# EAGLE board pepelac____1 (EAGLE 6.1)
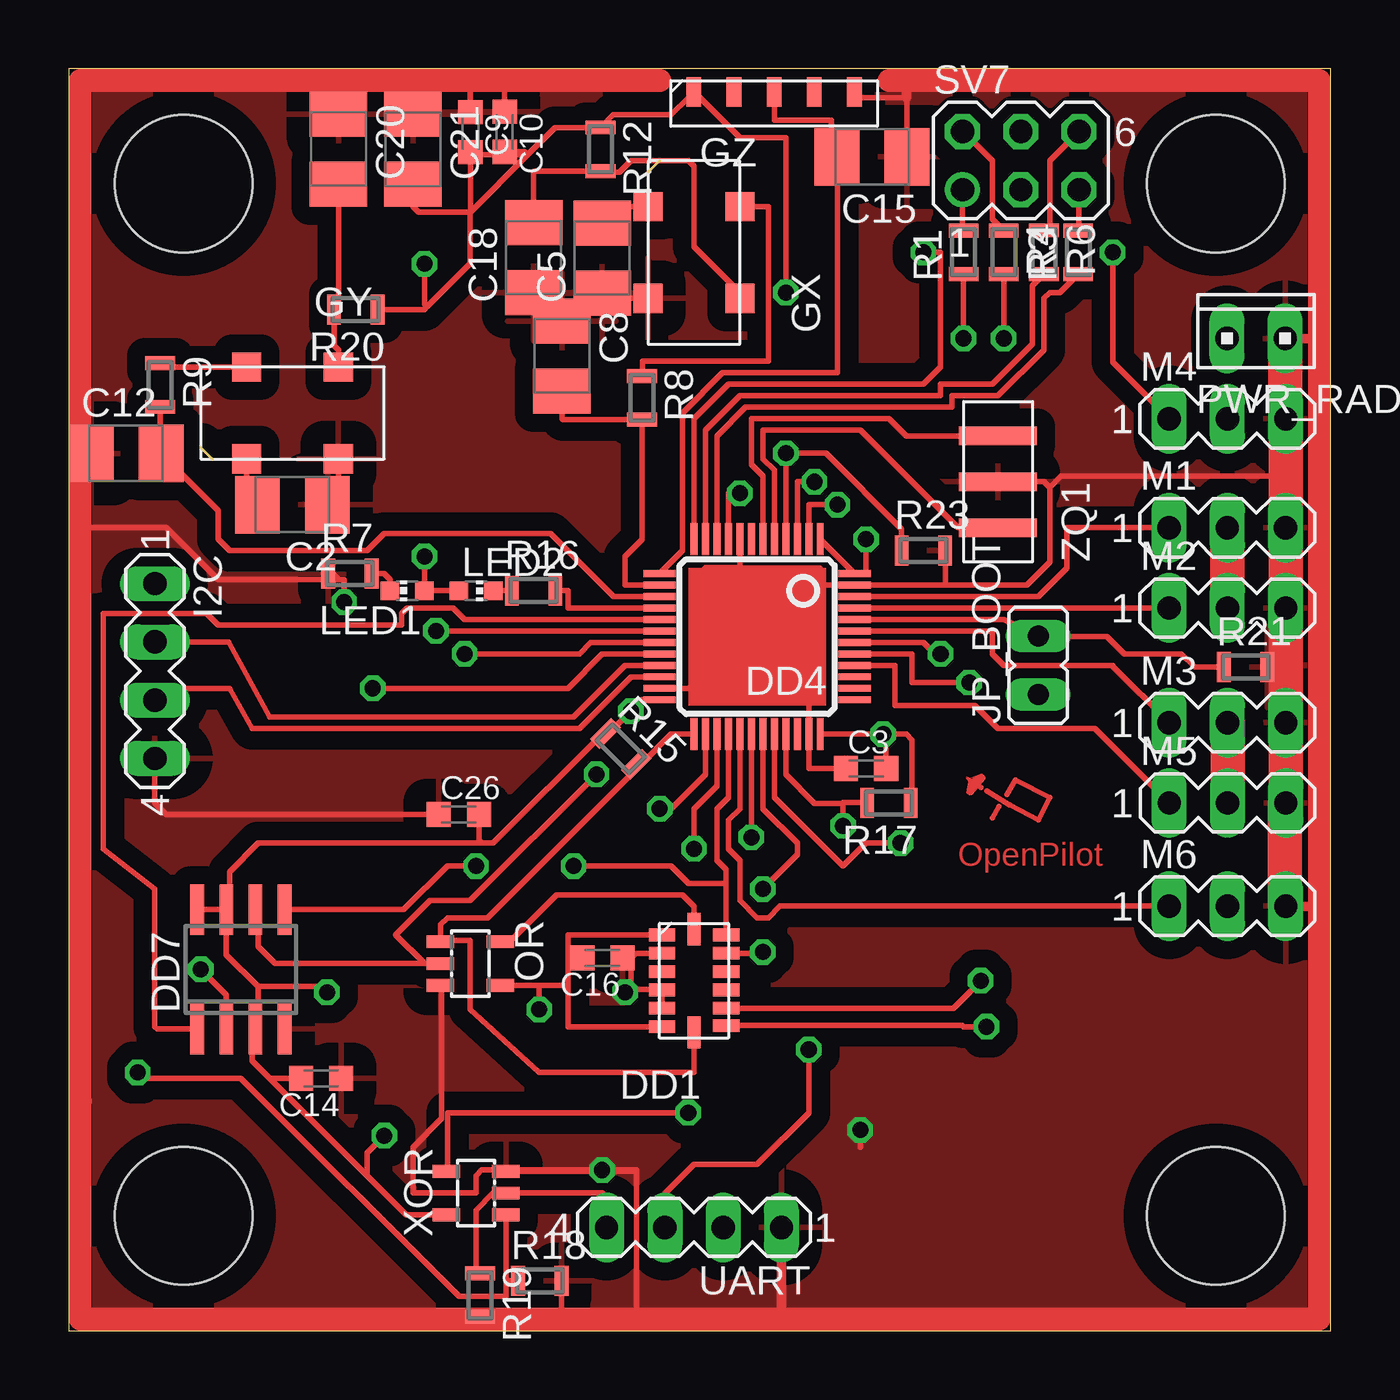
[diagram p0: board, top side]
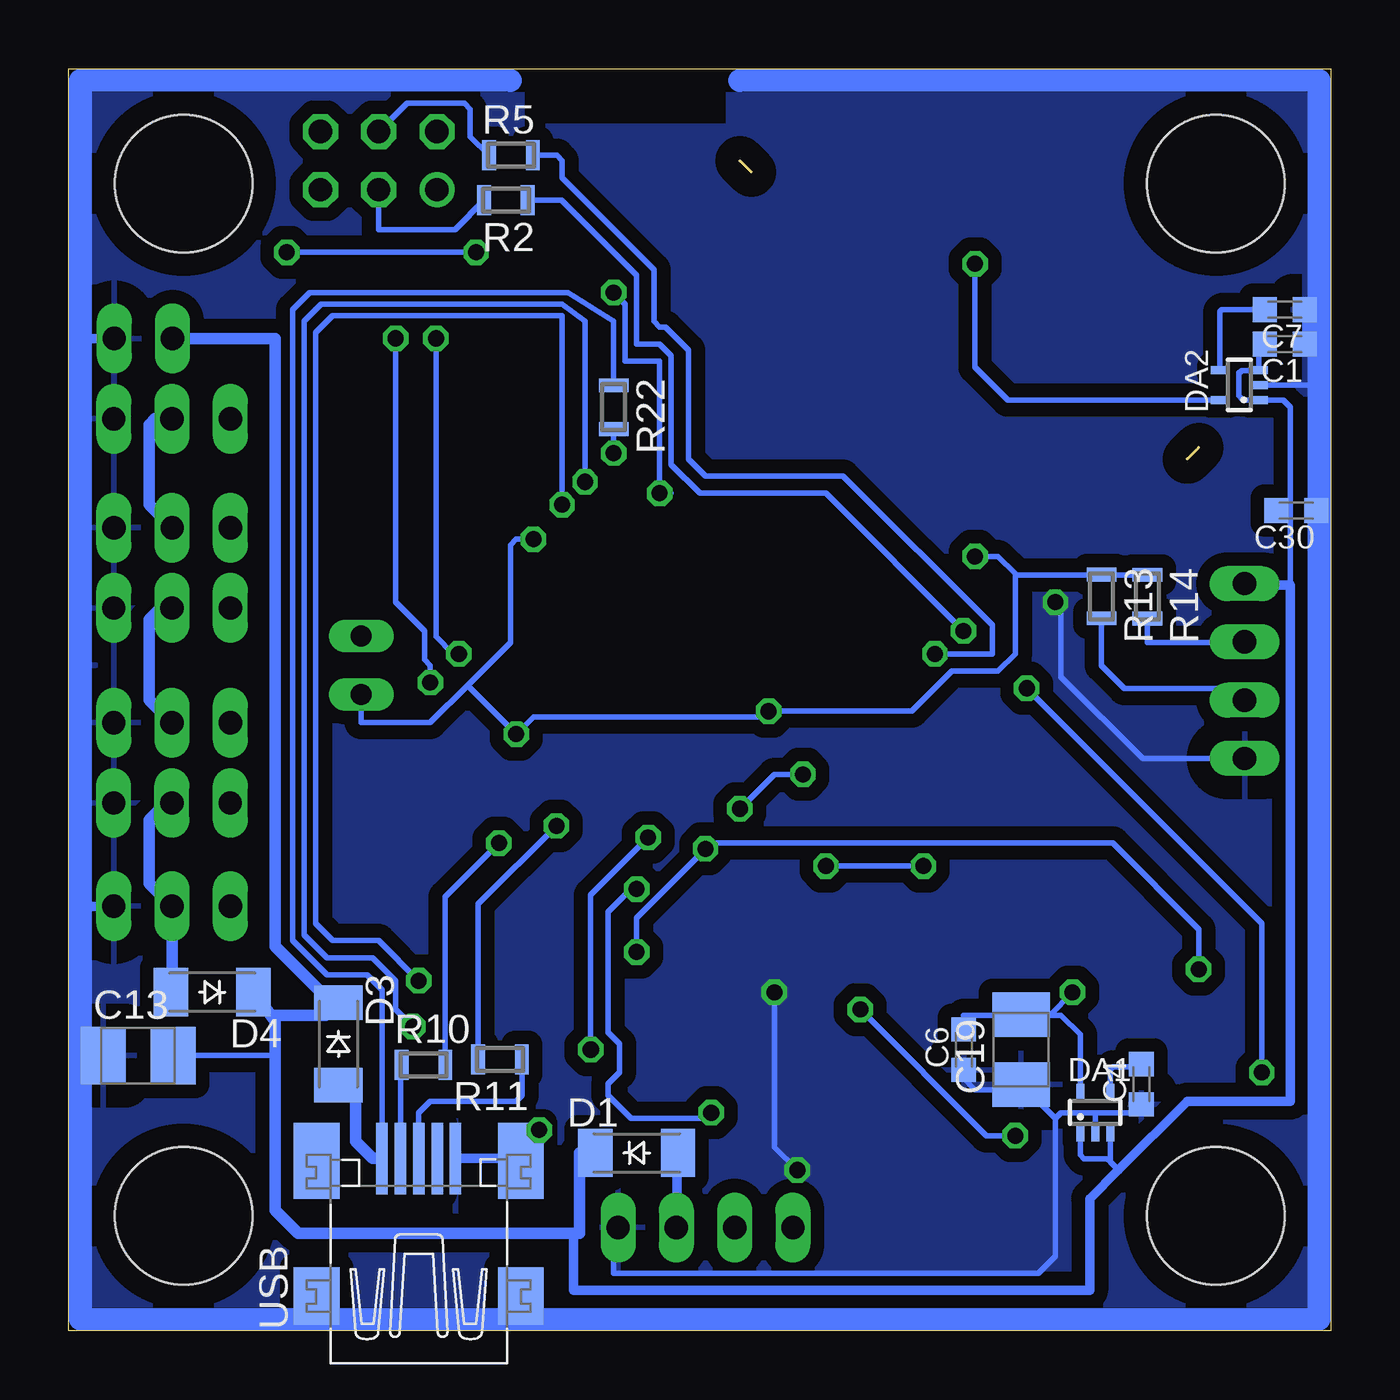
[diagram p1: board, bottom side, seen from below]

Size 55 x 55 mm. Coordinates in mm from the lower left corner, seen from the top.
Outline: 0,0 55,0 55,55 0,55 0,0
Copper layers (1*16): Top 0.035mm / dielectric 1.5mm / Bottom 0.035mm
Design rules: minimum track width 6mil, minimum drill 30mil, track to track 6mil, track to pad 6mil, pad to pad 8mil, via to via 8mil, smd to smd 8mil, copper to edge 40mil, drill to drill 8mil, minimum pad ring 10mil, minimum via ring 8mil, stop-mask expansion 4mil, vias tented up to drill 0mil, thermal gap 40mil
Holes 6 mm at 5,50 5,5 50,5 50,50

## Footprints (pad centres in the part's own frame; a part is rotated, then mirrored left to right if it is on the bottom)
C0603K = smd 1.05 x 1.08: 1 -0.875,0; 2 0.875,0
B/3528-21R = smd 1.95 x 2.5: + 1.525,0; - -1.525,0
SOD-123_MINI-SMA = smd 1.5 x 2.1: A 1.8,0; C -1.8,0
SC70-5L = smd 0.35 x 0.8: 1 -0.65,-0.85; 2 0,-0.85; 3 0.65,-0.85; 4 0.65,0.85; 5 -0.65,0.85
ACC = smd 1.145 x 0.55: 1 -1.4,2; 2 -1.4,1.2; 3 -1.4,0.4; 4 -1.4,-0.4; 5 -1.4,-1.2; 6 -1.4,-2; 8 1.4,-1.95; 9 1.4,-1.2; 10 1.4,-0.4; 11 1.4,0.4; 12 1.4,1.2; 13 1.4,2 | smd 0.55 x 1.4: 7 0,-2.25; 14 0,2.25
LQFP48 = smd 0.3 x 1.4: 1 -2.75,-4.25; 2 -2.25,-4.25; 3 -1.75,-4.25; 4 -1.25,-4.25; 5 -0.75,-4.25; 6 -0.25,-4.25; 7 0.25,-4.25; 8 0.75,-4.25; 9 1.25,-4.25; 10 1.75,-4.25; 11 2.25,-4.25; 12 2.75,-4.25; 25 2.75,4.25; 26 2.25,4.25; 27 1.75,4.25; 28 1.25,4.25; 29 0.75,4.25; 30 0.25,4.25; 31 -0.25,4.25; 32 -0.75,4.25; 33 -1.25,4.25; 34 -1.75,4.25; 35 -2.25,4.25; 36 -2.75,4.25 | smd 1.4 x 0.3: 13 4.25,-2.75; 14 4.25,-2.25; 15 4.25,-1.75; 16 4.25,-1.25; 17 4.25,-0.75; 18 4.25,-0.25; 19 4.25,0.25; 20 4.25,0.75; 21 4.25,1.25; 22 4.25,1.75; 23 4.25,2.25; 24 4.25,2.75; 37 -4.25,2.75; 38 -4.25,2.25; 39 -4.25,1.75; 40 -4.25,1.25; 41 -4.25,0.75; 42 -4.25,0.25; 43 -4.25,-0.25; 44 -4.25,-0.75; 45 -4.25,-1.25; 46 -4.25,-1.75; 47 -4.25,-2.25; 48 -4.25,-2.75
SOIC8 = smd 0.6 x 2.2: 1 -1.905,-2.6; 2 -0.635,-2.6; 3 0.635,-2.6; 4 1.905,-2.6; 5 1.905,2.6; 6 0.635,2.6; 7 -0.635,2.6; 8 -1.905,2.6
GIRO = smd 1.27 x 1.27: 1 1,2; 2 -3,2; 3 -3,-2; 4 1,-2
GZ = smd 0.635 x 1.27: 1 -3.5,0.5; 2 -1.75,0.5; 3 0,0.5; 4 1.75,0.5; 5 3.5,0.5
MA04-1 = drill 1.016 long: 1 -3.81,0; 2 -1.27,0; 3 1.27,0; 4 3.81,0
JP1 = drill 0.914 long: 1 0,-1.27; 2 0,1.27
CHIP-LED0603 = smd 0.8 x 0.8: A 0,-0.75; C 0,0.75
MA03-1 = drill 1.016 long: 1 -2.54,0; 2 0,0; 3 2.54,0
SOT23-5L = smd 0.55 x 1.2: 1 -0.95,-1.3; 2 0,-1.3; 3 0.95,-1.3; 4 0.95,1.3; 5 -0.95,1.3
10X02MTA = drill 1.016 long: 1 1.27,0; 2 -1.27,0
MINI_MELF-0102W = smd 0.6 x 1.3: 1 -0.95,0; 2 0.95,0
MA03-2 = drill 1.016: 1 -2.54,-1.27 | drill 1.016 octagon: 2 -2.54,1.27; 3 0,-1.27; 4 0,1.27; 5 2.54,-1.27; 6 2.54,1.27
32005-400 = smd 3.1 x 0.5: 1 3,1.6; 2 3,0.8; 3 3,0; 4 3,-0.8; 5 3,-1.6 | smd 2.5 x 2: M1 -3,-4.45; M2 -3,4.45 | smd 3.3 x 2: M3 2.9,4.45; M4 2.9,-4.45
QARZ = smd 0.8 x 3.4: 1 -2,0; 2 0,0; 3 2,0

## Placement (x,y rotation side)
C1  [C0603K]  2,43 180 bottom
C2  [B/3528-21R]  9.75,36 180 top
C3  [C0603K]  34.75,24.5 0 top
C4  [C0603K]  8.26,10.74 90 bottom
C5  [B/3528-21R]  23.25,46.75 90 top
C6  [C0603K]  15.99,12.25 90 bottom
C7  [C0603K]  2,44.5 180 bottom
C8  [B/3528-21R]  21.49,42.48 270 top
C9  [C0603K]  17.5,52.24 270 top
C10  [C0603K]  19,52.25 270 top
C12  [B/3528-21R]  2.5,38.24 0 top
C13  [B/3528-21R]  51.98,11.99 0 bottom
C14  [C0603K]  11,11 180 top
C15  [B/3528-21R]  35.01,51.16 180 top
C16  [C0603K]  23.25,16.25 180 top
C18  [B/3528-21R]  20.26,46.77 90 top
C19  [B/3528-21R]  13.5,12.25 90 bottom
C20  [B/3528-21R]  11.75,51.5 270 top
C21  [B/3528-21R]  15,51.49 270 top
C26  [C0603K]  17,22.5 0 top
C30  [C0603K]  1.5,35.75 180 bottom
D1  CGRM4001-G  [SOD-123_MINI-SMA]  30.25,7.75 0 bottom
D3  CGRM4001-G  [SOD-123_MINI-SMA]  43.25,12.5 270 bottom
D4  CGRM4001-G  [SOD-123_MINI-SMA]  48.75,14.75 180 bottom
DA1  [SC70-5L]  10.26,9.51 0 bottom
DA2  [SC70-5L]  3.98,41.22 90 bottom
DD1  [ACC]  27.25,15.25 0 top
DD4  [LQFP48]  30,30.25 180 top
DD7  [SOIC8]  7.5,15.75 0 top
GX  [GIRO]  27.25,47.99 90 top
GY  [GIRO]  8.75,40 180 top
GZ  [GZ]  30.74,53.49 0 top
I2C  [MA04-1]  3.75,28.75 270 top
JP_BOOT  [JP1]  42.25,29 0 top
LED1  [CHIP-LED0603]  14.75,32.25 90 top
LED2  [CHIP-LED0603]  17.75,32.25 270 top
M1  [MA03-1]  50.5,35 0 top
M2  [MA03-1]  50.5,31.5 0 top
M3  [MA03-1]  50.5,26.5 0 top
M4  [MA03-1]  50.5,39.75 0 top
M5  [MA03-1]  50.51,23 0 top
M6  [MA03-1]  50.5,18.5 0 top
OR  [SOT23-5L]  17.5,16 270 top
PWR_RADIO  [10X02MTA]  51.75,43.25 0 top
R1  [MINI_MELF-0102W]  39,47 90 top
R2  [MINI_MELF-0102W]  35.95,49.27 180 bottom
R3  [MINI_MELF-0102W]  44,47 90 top
R4  [MINI_MELF-0102W]  40.75,47 270 top
R5  [MINI_MELF-0102W]  35.73,51.23 0 bottom
R6  [MINI_MELF-0102W]  42.5,47.01 270 top
R7  [MINI_MELF-0102W]  12.25,33 0 top
R8  [MINI_MELF-0102W]  24.98,40.66 270 top
R9  [MINI_MELF-0102W]  3.98,41.22 270 top
R10  [MINI_MELF-0102W]  39.54,11.59 0 bottom
R11  [MINI_MELF-0102W]  36.21,11.83 180 bottom
R12  [MINI_MELF-0102W]  23.17,51.49 270 top
R13  [MINI_MELF-0102W]  9.99,32 270 bottom
R14  [MINI_MELF-0102W]  8,31.99 270 bottom
R15  [MINI_MELF-0102W]  24.06,25.36 315 top
R16  [MINI_MELF-0102W]  20.26,32.25 0 top
R17  [MINI_MELF-0102W]  35.75,23 180 top
R18  [MINI_MELF-0102W]  20.53,2.17 0 top
R19  [MINI_MELF-0102W]  17.92,1.55 270 top
R20  [MINI_MELF-0102W]  12.51,44.5 180 top
R21  [MINI_MELF-0102W]  51.29,28.92 0 top
R22  [MINI_MELF-0102W]  31.25,40.25 270 bottom
R23  [MINI_MELF-0102W]  37.25,34 0 top
SV7  [MA03-2]  41.49,51 0 top
UART  [MA04-1]  27.25,4.5 180 top
USB  MINI-USB_SHIELD5P4-32005-400  [32005-400]  39.75,4.5 90 bottom
XOR  SN74LVC1G86DBVR  [SOT23-5L]  17.75,6 90 top
ZQ1  QARZ  [QARZ]  40.5,37 90 top

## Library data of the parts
C1 C3 C4 C6 C7 C9 C10 C14 C16 C26 C30 R1-R23 = resistor
C2 C5 C8 C12 C13 C15 C18-C21 = rcl
D1 D3 D4 = diode
DA1 DA2 DD1 DD4 DD7 GX GY GZ OR XOR ZQ1 = pepelac
I2C M1-M6 SV7 UART = con-lstb; OC_FARNELL: unknown; OC_NEWARK: unknown
JP_BOOT = jumper
LED1 LED2 = led
PWR_RADIO = con-amp
USB = con-cypressindustries; OC_FARNELL: unknown; OC_NEWARK: unknown

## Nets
+5V: D4.A M1.2 M2.2 M3.2 M4.2 M5.2 M6.2
GND: C1.1 C2.- C3.1 C4.1 C5.- C6.1 C7.1 C8.- C9.1 C10.1 C12.- C13.- C14.1 C15.- C16.1 C18.- C19.- C20.- C21.- C26.1 C30.1 DA1.2 DA2.2 DD1.2 DD1.4 DD1.5 DD4.8 DD4.23 DD4.35 DD4.47 DD7.4 GX.2 GY.2 GZ.5 I2C.4 M1.3 M2.3 M3.3 M4.3 M5.3 M6.3 OR.3 PWR_RADIO.1 R7.1 R18.2 R19.2 R21.2 R23.2 UART.1 USB.5 XOR.3 ZQ1.2
N$1: DD4.6 ZQ1.3
N$2: GX.4 R8.1
N$3: GY.4 R9.1
N$4: DD1.7 DD4.25 OR.1 R15.2
N$5: DD4.16 R16.2
N$6: DD4.33 R11.2 R17.2
N$7: DD4.29 M6.1
N$8: D1.A UART.2
N$9: C18.+ GX.3 R12.2
N$10: C20.+ GY.3 R20.2
N$11: DD1.9 DD4.2
N$12: LED2.C R16.1
N$13: C7.2 DA2.4
N$14: C12.+ DD4.15 R9.2
N$15: C8.+ DD4.14 R8.2
N$16: LED1.C R7.2
N$17: DD1.8 DD4.3
N$18: C2.+ GY.1
N$19: R1.2 SV7.1
N$20: R2.2 SV7.3
N$21: R3.2 SV7.5
N$22: R4.1 SV7.2
N$23: R5.1 SV7.4
N$24: R6.1 SV7.6
N$25: DD4.42 R1.1
N$26: DD4.41 R4.2
N$27: DD4.18 R2.1
N$28: DD4.19 R5.2
N$29: DD4.10 R3.1
N$30: DD4.11 R6.2
N$31: C15.+ DD4.13 GZ.3
N$32: DD4.5 ZQ1.1
N$34: DD4.46 M1.1
N$35: DD4.45 M2.1
N$36: DD4.43 M3.1
N$37: DD4.40 M5.1
N$38: DD4.12 M4.1
N$39: C5.+ GX.1
N$40: R19.1 UART.4 XOR.2
N$41: C4.2 DA1.4
N$43: DD4.30 UART.3
N$44: DD4.4 R22.2 R23.1
N$45: D3.A R22.1 USB.1
N$46: R10.1 USB.2
N$47: R11.1 USB.3
N$48: DD4.20 R18.1 XOR.1
N$49: DD4.31 XOR.4
N$50: DD4.22 I2C.3 R13.2
N$51: DD4.21 I2C.2 R14.2
N$53: DD4.32 R10.2
N$54: DD4.44 JP_BOOT.2 R21.1
N$58: DD4.17 DD7.1
N$60: DD4.26 DD7.6 OR.2
N$61: DD1.12 DD4.27 DD7.2
N$62: DD1.14 OR.5
N$63: DD1.13 DD4.28 DD7.5
V+: C1.2 C13.+ C30.2 D1.C D3.C D4.C DA1.1 DA1.3 DA2.1 DA2.3 PWR_RADIO.2
VCC: C9.2 C10.2 C21.+ DA2.5 DD4.9 GZ.1 R12.1 R20.1
VDD: C3.2 C6.2 C14.2 C16.2 C19.+ C26.2 DA1.5 DD1.1 DD1.6 DD4.1 DD4.24 DD4.36 DD4.48 DD7.3 DD7.7 DD7.8 JP_BOOT.1 LED1.A LED2.A OR.4 R13.1 R14.1 R15.1 R17.1 XOR.5

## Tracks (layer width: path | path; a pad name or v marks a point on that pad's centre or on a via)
+5V  (via drill 0.7)
  Top 0.5: M3.2
  Top 1.5: M4.2 | M1.2 M2.2 M1.2 | M3.2 M5.2
  Bottom 0.5: M4.2 51.25,39.75 51.5,39.5 51.5,36 M1.2 | M2.2 51,31.5 51.5,31 51.5,27.5 M3.2 | M5.2 50.75,23 51.5,22.25 51.5,19.5 M6.2 50.5,14.8 D4.A
  other vias: 50.5,31.5
GND  (via drill 0.7)
  Top 0.25: ZQ1.2 42.5,37 42.75,36.75 | 42.75,36.75 42.75,33.5 41.75,32.5 39.75,32.5 | 39.75,32.5 DD4.47 32.75,32.5 | 42.75,36.75 43.25,37.25 53,37.25 53,35 | 32.75,32.5 32.75,33.25 29.25,33.25 | 29.25,33.25 DD4.8 | DD4.23 27,28 27.25,28.25 27.25,32.75 27.75,33.25 29.25,33.25 | 32.75,32.5 32.25,32.5 DD4.35 32.25,24.5 | GZ.5 34.48,53.75 36.5,53.75 36.53,53.72 C15.- | DD1.2 24.7,16.45 24.5,16.25 | 24.5,16.25 24.5,15 | 24.5,15 24.5,14.99 24.61,14.88 25.82,14.88 DD1.4 | DD1.4 DD1.5 DD1.4 | 0.75,10.25 0.5,10 | R23.2 38.2,32.55 38.25,32.5 39.75,32.5 | 39.75,32.5 | 24.5,15 v24.25,14.75 24.38,14.88 26.05,14.88 26,14.93 26,15 DD1.4 | XOR.3 24.7,6.95 24.75,7 | 24.75,7 24.75,0.5 | 24.75,7 v23.25,7 18,7 17.75,6.75 17.75,6 15,6 15,8 16.25,9.25 16.25,15 OR.3 | 12,37.75 GY.2 | v34.5,8.75 34.5,8 | R19.2 18.9,0.6 19,0.5 | R21.2 52.96,28.92 53.04,29 | GX.2 23.47,44.99 C5.- 22.71,45.22 C8.- C18.- | v12,31.75 12,32.75 11.75,32.75 | 11.75,32.75 6.5,32.75 4.25,35 0.5,35 | C12.- 0.51,38.24 0.5,38.25 | C2.- 11.5,36 11.75,36.25 GY.2 | C21.- 15,54.25 17.5,54.25 C9.1 | 17.5,53 C9.1 | C9.1 | R7.1 11.5,33 11.75,32.75 | R18.2 21.48,0.77 21.75,0.5 | C3.1 32.25,24.5 | 32.25,24.5 | C10.1 19,54.25 19.25,54.5 | C16.1 24.5,16.25 | C26.1 4.25,22.5 3.75,23 3.75,25
  Top 0.406: 36.5,53.75 36.5,54.5 | 35.75,54.5 54.5,54.5 54.5,43.5 54.25,43.25 v53,43.25 | UART.1 31.06,0.69 31.25,0.5 | 53.25,18.5 54.5,18.5
  Top 1: 35.75,54.5 36.5,54.5 54.5,54.5 54.5,18.5 54.5,0.5 31.25,0.5 24.75,0.5 21.75,0.5 19,0.5 0.5,0.5 0.5,10 0.5,35 0.5,38.25 0.5,54.5 19.25,54.5 25.75,54.5
  Top 1.5: M6.3 53,18.5 53,23 | M5.3 M3.3 53.04,29 M2.3 M1.3 | 53,35 M1.3 M4.3 53.02,39.75 PWR_RADIO.1
  Bottom 0.25: v24.25,14.75 24.25,8 v23.25,7 | I2C.4 8.19,24.94 11.75,28.5 11.75,31.25 v12,31.75 | 35.5,7.5 34.5,7.5 v34.5,8.75 | DA2.2 0.53,41.22 0.5,41.25 | DA1.2 10.26,9.49 10.25,9.5 | 10.25,9.5 11.75,9.5 12,9.25 | 12,9.25 12,3.25 12.75,2.5 31.25,2.5 31.25,4.25 31,4.5 | C4.1 8.38,9.87 8.75,9.5 10.25,9.5 | C30.1 0.5,35.75 | 12,9.25 13.48,10.73 C19.- 13.73,10.5 15.5,10.5 15.99,10.99 C6.1 | C13.- 54.49,11.99 54.5,12 | C7.1 C1.1 1,43 0.5,42.5
  Bottom 0.406: USB.5 35.5,7.5 | v53,43.25 54.5,43.25 | 53,18.5 54.5,18.5
  Bottom 1: 35.75,54.5 54.5,54.5 54.5,43.25 54.5,18.5 54.5,12 54.5,0.5 0.5,0.5 0.5,35.75 0.5,41.25 0.5,42.5 0.5,54.5 25.75,54.5
  pour Top (isolate 0.8): 0,55 26.25,55 26.25,54.75 26.25,52.5 35.25,52.5 35.25,55 55,55 55,0 0,0
  pour Bottom (isolate 0.6): 26.25,55 26.25,52.5 35.25,52.5 35.25,55 55,55 55,0 0,0 0,55
N$1
  Top 0.25: DD4.6 30.25,36 30.25,37.25 29.75,37.75 29.75,39.75 35.75,39.75 36.5,39 ZQ1.3 | 40.75,39 ZQ1.3 | ZQ1.3
N$2
  Top 0.152: 25,41.75 R8.1
  Top 0.25: GX.4 30.5,48.99 30.5,49 30.5,42.25 25,42.25 25,41.75 25,41.5
N$3
  Top 0.25: GY.4 4.15,42 R9.1
N$4
  Top 0.25: DD1.7 27.25,11.25 20.5,11.25 17.5,14 17.5,17 16.25,17 OR.1 16.2,17.7 16.5,18 18.25,18 24.94,24.69 | DD4.25 26.25,26 24.94,24.69 | R15.2 24.94,24.69
N$5
  Top 0.152: 21.25,32.25 R16.2
  Top 0.25: DD4.16 21.75,31.5 21.75,32.25 21.25,32.25
N$6  (via drill 0.7)
  Top 0.25: v33.75,22 33.75,23.02 | DD4.33 31.25,24.25 32.49,22.99 33.72,22.99 33.75,23.02 | 33.75,23.02 34.78,23.02 R17.2
  Bottom 0.25: R11.2 37.16,18.59 v33.75,22
N$7
  Top 0.25: M6.1 31,18.5 30.5,18 30,18 29.25,18.75 29.25,20.5 28.75,21 28.75,22.25 29.25,22.75 DD4.29
N$8
  Bottom 0.152: 28.5,7.75 D1.A
  Bottom 0.406: UART.2 28.5,4.5 28.5,7.75
N$9
  Top 0.25: GX.3 29.25,45.25 27.25,47.25 27.25,50.75 27,51 24.5,51 24,50.5 23.21,50.5 R12.2 20.29,50.54 20.25,50.5 20.25,48.3 C18.+
N$10
  Top 0.152: 11.5,44.5 R20.2
  Top 0.25: R20.2 11.56,42.94 11.75,42.75 GY.3 | C20.+ 11.75,44.75 11.5,44.5
N$11  (via drill 0.7)
  Top 0.25: DD4.2 32.25,36 v33.5,36 | v39.75,15.25 38.55,14.05 DD1.9
  Bottom 0.25: v33.5,36 33.5,44.25 43.5,44.25 44.25,43.5 44.25,17.75 43.5,17 41.5,17 v39.75,15.25
N$12
  Top 0.25: LED2.C R16.1
N$13
  Bottom 0.152: 3,44.5 C7.2
  Bottom 0.25: DA2.4 4.83,44.42 4.75,44.5 3,44.5
N$14
  Top 0.25: R9.2 3.98,38.28 C12.+ 4.02,38.23 6.5,35.75 6.5,34.5 7,34 13,34 13.75,34.75 21,34.75 23.75,32 DD4.15
N$15
  Top 0.25: C8.+ 21.5,39.75 21.54,39.71 R8.2 24.98,34.48 24.25,33.75 24.25,32.5 DD4.14
N$16
  Top 0.152: LED1.C
  Top 0.25: R7.2 13.75,33 14,32.75 LED1.C
N$17  (via drill 0.7)
  Top 0.25: DD4.3 31.75,36 31.75,37 v32.5,37 | v40,13.25 39,13.25 38.95,13.3 DD1.8
  Bottom 0.25: v32.5,37 32.5,44 33.5,44.75 44,44.75 44.75,44 44.75,17.25 43.75,16.25 41.75,16.25 40.75,15.25 40.75,14 v40,13.25
N$18
  Top 0.25: C2.+ 7.75,36 GY.1
N$19
  Top 0.25: R1.2 38.95,48 SV7.1
N$20
  Bottom 0.25: R2.2 38.17,48 41.5,48 41.49,48.01 SV7.3
N$21
  Top 0.25: R3.2 44.03,47.99 SV7.5
N$22
  Top 0.25: R4.1 40.25,48.45 40.25,51 38.98,52.27 SV7.2
N$23
  Bottom 0.152: 41.5,52.25 SV7.4
  Bottom 0.25: R5.1 37.5,52.05 37.5,53.25 37.75,53.5 40.25,53.5 41.5,52.25
N$24
  Top 0.25: R6.1 42.75,48.2 42.75,51 44.02,52.27 SV7.6
N$25  (via drill 0.7)
  Top 0.25: v39,43.25 R1.1 | DD4.42 37.25,30 37.75,29.5 v38,29.5
  Bottom 0.25: v39,43.25 39,30.25 38.25,29.5 v38,29.5
N$26  (via drill 0.7)
  Top 0.152: 40.75,46 R4.2
  Top 0.25: v40.75,43.25 40.75,46 | DD4.41 36.75,29.5 36.75,28.25 v39.25,28.25
  Bottom 0.25: v40.75,43.25 40.75,31.75 39.5,30.5 39.5,29.25 39.25,29 v39.25,28.25
N$27  (via drill 0.7)
  Top 0.25: DD4.18 v16,30.5
  Bottom 0.25: R2.1 33.52,49.27 30.25,46 30.25,43 29.25,43 28.75,42.5 28.75,37.75 27.5,36.5 22,36.5 v16,30.5
N$28  (via drill 0.7)
  Top 0.25: DD4.19 22.75,30 22.25,29.5 v17.25,29.5
  Bottom 0.25: R5.2 33.73,51.23 33.5,51 33.5,50.25 29.5,46.25 29.5,44 29.25,43.75 29,43.75 28,42.75 28,38 27.25,37.25 21.25,37.25 14.75,30.75 14.75,29.5 v17.25,29.5
N$29
  Top 0.152: DD4.10
  Top 0.25: R3.1 43.2,45.25 42.75,45.25 42.5,45 42.5,42.75 40.5,40.75 38.5,40.75 38.5,40.25 29.5,40.25 28.25,39 DD4.10
N$30
  Top 0.25: R6.2 42,45.55 42,43 40.25,41.25 38,41.25 38,40.75 29.25,40.75 27.75,39.25 DD4.11 | DD4.11 27.75,34.25 | DD4.11
N$31
  Top 0.152: 30.75,53.75 GZ.3
  Top 0.25: DD4.13 26.75,34 26.75,40 28.5,41.75 33.5,41.75 33.5,51.15 | GZ.3 30.75,53.75 30.75,52.75 33.25,52.75 33.25,51.5 33.5,51.25 33.5,51.15 | C15.+ 33.5,51.15
N$32
  Top 0.25: DD4.5 30.75,36.25 30.75,37.5 30.25,38 30.25,39.25 34.5,39.25 38.75,35 ZQ1.1
N$34
  Top 0.25: M1.1 43.5,35 43.5,33.25 42.25,32 DD4.46
N$35
  Top 0.25: M2.1 48,31.5 42.75,31.5 DD4.45
N$36
  Top 0.152: DD4.43
  Top 0.25: DD4.43 40.25,30.5 40.25,29.5 40.75,29 45.5,29 45.5,28.96 M3.1
N$37
  Top 0.152: DD4.40
  Top 0.25: M5.1 44.72,26.25 40.5,26.25 39.5,27.25 36,27.25 36,29 DD4.40
N$38  (via drill 0.7)
  Top 0.152: 27.25,34.75 DD4.12
  Top 0.25: M4.1 45.5,42.21 v45.5,47 | 27.25,34.75 27.25,39.75 28.75,41.25 37.25,41.25 38,42 38,47 v37.25,47
  Bottom 0.25: v45.5,47 v37.25,47
N$39
  Top 0.25: C5.+ 23.25,48.99 23.25,49 GX.1
N$40
  Top 0.152: 18,2.5 R19.1
  Top 0.25: UART.4 23.44,5.81 23.25,6 XOR.2 | XOR.2 | XOR.2 18.5,6 17.75,5.25 17.75,2.75 18,2.5
N$41
  Bottom 0.25: DA1.4 9.61,11.39 9.5,11.5 8.25,11.5 C4.2
N$43  (via drill 0.7)
  Top 0.25: UART.3 25.98,5.98 27.25,7.25 30,7.25 32.25,9.5 v32.25,12.25 | v29.75,21.5 DD4.30
  Bottom 0.25: v32.25,12.25 32.25,19 v29.75,21.5
N$44  (via drill 0.7)
  Top 0.152: DD4.4
  Top 0.25: DD4.4 v31.25,38.25 33,38.25 36.3,34.95 R23.1
  Bottom 0.25: R22.2 v31.25,38.25
N$45
  Bottom 0.25: USB.1 41.35,14.85 42,15.5 43.75,15.5 45.25,17 45.25,44.5 44.5,45.25 33.25,45.25 31.25,44 R22.1
  Bottom 0.5: USB.1 41.75,7.5 42.5,8.25 42.5,10.75 43.2,10.75 D3.A
N$46
  Bottom 0.25: USB.2 40.55,11.53 R10.1
N$47
  Bottom 0.152: 35.25,11.75 R11.1
  Bottom 0.25: USB.3 39.75,9.5 39.25,10 35.5,10 35.25,10.25 35.25,11.75
N$48  (via drill 0.7)
  Top 0.25: DD4.20 23.5,29.5 23.25,29.5 21.75,28 v13.25,28 | XOR.1 19.05,3.8 19.06,2.23 | 19.06,2.23 19.06,1.49 17,1.5 7.5,11 3.25,11 v3,11.25 | R18.1 19.16,2.17 19.09,2.23 19.06,2.23 | 19.06,2.23
  Bottom 0.25: v3,11.25 3,17.75 v13.25,28
N$49  (via drill 0.7)
  Top 0.152: 16.5,7 XOR.4
  Top 0.25: DD4.31 30.25,22.75 31.75,21.25 31.75,20.75 v30.25,19.25 | v27,9.5 16.5,9.5 16.5,7
  Bottom 0.25: v30.25,19.25 30.5,19.25 31.5,18.25 31.5,13 31,12.5 31,11.25 31.5,10.75 31.5,10.25 30.5,9.25 27,9.25 v27,9.5
N$50
  Top 0.25: DD4.22 24.5,28.5 22.25,26.25 8,26.25 7,28 4.25,28 3.75,27.5 I2C.3
  Bottom 0.25: R13.2 9.99,28.99 9,28 3.75,28 I2C.3
N$51
  Top 0.25: DD4.21 24.25,29 22,26.75 8.75,26.75 6.98,30.02 I2C.2
  Bottom 0.152: 3.75,30 I2C.2
  Bottom 0.25: 3.79,30.04 3.75,30 8,30 R14.2
N$53  (via drill 0.7)
  Top 0.25: v36.25,21.25 34.75,21.25 33.75,20.25 30.75,23.25 DD4.32
  Bottom 0.25: R10.2 38.59,18.91 v36.25,21.25
N$54
  Top 0.152: 42.5,30.25 JP_BOOT.2
  Top 0.25: JP_BOOT.2 40.75,31 DD4.44 | R21.1 49.08,28.92 48.5,29.5 46,29.5 45.25,30.25 42.5,30.25 42.25,30.25
N$58
  Top 0.25: DD4.17 17.25,31 16.75,31.5 14.75,31.5 14.5,31.25 14.5,30.75 6.5,30.75 6,31.25 1.5,31.25 1.5,21 3.75,19.25 3.75,13.25 3.85,13.15 DD7.1
N$60  (via drill 0.7)
  Top 0.25: v23,24.25 17.5,18.75 15.75,18.75 14.25,17.25 15.5,16 OR.2 9,16 8.25,16.75 8.25,18.23 DD7.6 | v25.75,22.75 26.25,22.75 27.75,24.25 DD4.26
  Bottom 0.25: v23,24.25 24.25,24.25 v25.75,22.75
N$61  (via drill 0.7)
  Top 0.25: DD1.12 30.2,16.45 v30.25,16.5 | v27.25,21 27.25,22.75 28.25,23.75 DD4.27 | DD7.2 6.86,14.64 v5.75,15.75
  Bottom 0.25: v30.25,16.5 30.25,18 v27.25,21 27,21.25 9.5,21.25 5.75,17.5 v5.75,15.75
N$62
  Top 0.25: OR.5 19.2,16.95 21.25,19 26.75,19 27.25,18.5 DD1.14
N$63  (via drill 0.7)
  Top 0.25: DD1.13 28.65,19.5 | 28.65,19.5 28.65,20.1 28.25,20.5 28.25,22.75 28.75,23.25 DD4.28 | DD7.5 14.6,18.35 16.5,20.25 v17.75,20.25 | v22,20.25 26.25,20.25 27,19.5 28.65,19.5
  Bottom 0.25: v17.75,20.25 v22,20.25
S$1
  Top 0.25: 40.88,23.38 41.25,24 42.75,23.25 42.25,22.25 41.01,22.91
S$2
  Top 0.25: 39.75,23.68 39.36,23.95 39.55,23.83 39.78,24.13 39.44,23.99 39.35,23.89 39.26,23.51 39.26,23.5 39.62,23.92 39.84,24.09 39.32,23.45 39.5,24 39.5,23.75
S$3
  Top 0.09: 39.25,24 39.18,24.08 39.24,24.05 39.25,24
S$4
  Top 0.03: 39.91,24.17 39.79,24.26 39.24,24.04 39.13,23.45 39.26,23.36
S$5
  Top 0.03: 39.11,24.12 39.22,23.96 39.3,24.07 39.12,24.13
S$6
  Top 0.03: 39.72,23.61 39.81,23.72
S$7
  Top 0.25: 41,22.92 40.02,23.52
S$8
  Top 0.25: 40.53,22.84 40.25,22.34
V+
  Bottom 0.25: 1.75,35.75 1.75,40.25 2.07,40.57 DA2.1 3.82,40.57 4,40.75 4,41.75 3.97,41.75 3.87,41.85 3.15,41.85 DA2.3 3.13,42.75 C1.2 3,43 | 1.75,35.75 1.75,32.5 | DA1.3 9.61,7.36 | 9.61,7.36 9.25,7 | DA1.1 10.91,7.66 10.75,7.5 9.75,7.5 9.61,7.36 | C13.+ 46.01,11.99 46,12 | C30.2 1.75,35.75
  Bottom 0.406: 3.75,32.5 1.75,32.5 1.75,10 6.25,10 9.25,7 10.5,5.75 10.5,1.75 33,1.75 33,4.25
  Bottom 0.5: D1.C 32.75,7.75 32.75,4.25 33,4.25 45,4.25 46,5.25 46,12 46,13.5 | 46,13.5 46,13.75 43.8,13.75 D3.C 43.25,14.25 43.5,14.25 46,16.75 46,43.25 PWR_RADIO.2 | D4.C 46,13.5
VCC  (via drill 0.7)
  Top 0.152: 27,53.75 GZ.1
  Top 0.25: DD4.9 28.75,36.5 v29.25,36.5 | v31.25,45.25 31.25,52 29.25,52 GZ.1 27,53.75 26.25,53 23.73,53 R12.1 21.19,52.44 20,51.25 | 20,51.25 17.5,48.75 | 17.5,48.75 17.5,46.5 15.62,44.62 | 15.62,44.62 15.5,44.5 R20.1 | C21.+ 15,49 15.25,48.75 17.5,48.75 | v15.5,46.5 15.5,44.75 15.62,44.62 | C10.2 19.87,51.38 20,51.25 | 20,51.25 17.5,51.25 | C9.2 17.5,48.75 | 17.5,48.75
  Bottom 0.25: 28.75,36.5 v29.25,36.5 29.25,42.25 30.75,42.25 30.75,44.75 v31.25,45.25 | DA2.5 14.07,40.57 15.5,42 v15.5,46.5
VDD  (via drill 0.7)
  Top 0.152: DD4.1 | 7,18.5 DD7.7 | DD4.48
  Top 0.25: v34.75,34.5 34.75,33 DD4.48 DD4.1 | DD4.36 v35.5,26 | DD4.24 25,27.5 v24.5,27 23.53,26.03 R15.1 23.28,26.03 18.5,21.25 18,21.25 | DD1.1 21.75,17.25 21.75,16.25 | 21.75,16.25 21.75,15 | 21.75,15 21.75,13.25 DD1.6 | OR.4 20.5,15.05 | 20.5,15.05 21.7,15.05 21.75,15 | DD7.8 DD7.7 6.86,16.39 8.25,15 | 8.25,15 8.25,13.27 DD7.3 8,13.02 8,11.75 8.75,11 | 13,6.75 8.75,11 | XOR.5 14.7,5.05 13,6.75 | 13,6.75 13,7.75 v13.75,8.5 | v20.5,14 20.5,15.05 | LED2.A LED1.A v15.5,33.75 | 18,21.25 8.25,21.25 7,20 7,18.5 | R17.1 36.7,23.45 36.75,23.5 36.75,25.75 36.5,26 v35.5,26 | 35.59,25.91 v35.5,26 | C3.2 35.62,25.88 v35.5,26 | C14.2 8.75,11 | v11.25,14.75 11,15 8.25,15 | C16.2 21.75,16.25 | C26.2 17.87,21.38 18,21.25
  Bottom 0.152: 42.25,27.75 JP_BOOT.1
  Bottom 0.25: JP_BOOT.1 42.23,27.75 | 37.62,28.12 39.25,26.5 42.25,26.5 42.25,27.75 | 37.62,28.12 35.75,30 35.75,34.25 35.5,34.5 v34.75,34.5 | 37.62,28.12 v35.5,26 34.75,26.75 24.75,26.75 v24.5,27 18.25,27 16.5,28.75 14.5,28.75 13.75,29.5 13.75,31.75 | v13.75,8.5 15,8.5 v20.5,14 | 9.97,32.94 R13.1 | R14.1 9.97,32.94 | 9.97,32.94 13.75,32.93 13.75,31.75 | 13.75,31.75 13.75,33 14.5,33.75 v15.5,33.75 | 12.25,13.75 11.75,13.75 10.91,12.91 DA1.5 | 13.47,13.75 C19.+ 13.5,13.75 | C6.2 15.99,13.74 16,13.75 13.5,13.75 | 13.47,13.75 13.5,13.75 | 13.47,13.75 12.25,13.75 | 12.25,13.75 v11.25,14.75
(copper drawn outside any net)
  shapes: Top area x2

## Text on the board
Top: OpenPilot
